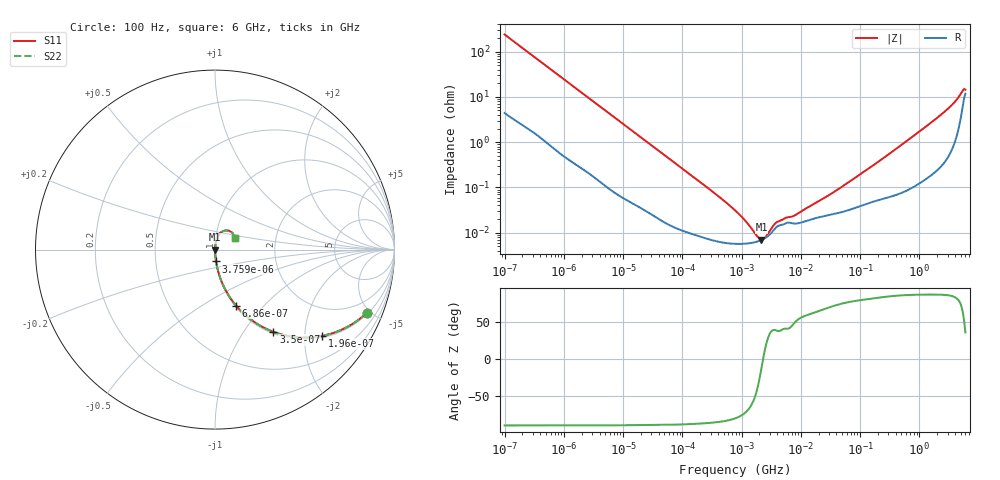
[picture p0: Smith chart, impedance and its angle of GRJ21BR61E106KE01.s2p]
!Murata Part Number: GRJ21BR61E106KE01
!These Parameters are Measured in Series Mode Connection
!Data Generated on Jun 19, 2026
!  o--ll--o
!Port1  Port2
!  o------o
!Operation Temp=25[degC], DC Bias Voltage=0[V]
!Freq. Start=100[Hz] Stop=6[GHz] 401[Steps]
# Hz S RI R 50
!Freq.(Hz) S11(Real) S11(Imag) S21(Real) S21(Imag) S12(Real) S12(Imag) S22(Real) S22(Imag)
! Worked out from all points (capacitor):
!   401 points, 100 Hz to 6 GHz, reference 50 ohm
!   read as one part in series: C = 6.67 uF near 109 Hz
!   lowest |Z| = 7.08 mohm at 2.169 MHz (marker M1)
!   series resonance near 2.31 MHz, so ESL is about 710 pH
!   S11 on the Smith chart (normalised r, x): 100 Hz: 1.09, -4.75; 196 Hz: 1.05, -2.45; 350 Hz: 1.03, -1.38; 686 Hz: 1.01, -0.71; 3.759 kHz: 1.00, -0.13; 6 GHz: 1.23, +0.17
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100  0.8451 -0.3526  0.1549 0.3526  0.1549 0.3526  0.8451 -0.3526
196  0.5976 -0.4805  0.4024 0.4805  0.4024 0.4805  0.5976 -0.4805
350  0.3256 -0.4583  0.6744 0.4583  0.6744 0.4583  0.3256 -0.4583
686  0.117 -0.3116  0.883 0.3116  0.883 0.3116  0.117 -0.3116
2008  0.0174 -0.1204  0.9826 0.1204  0.9826 0.1204  0.0174 -0.1204
3759  0.0058 -0.0658  0.9942 0.0658  0.9942 0.0658  0.0058 -0.0658
40335  0.00024 -0.00638  0.9998 0.00638  0.9998 0.00638  0.00024 -0.00638
330837  6.82e-05 -0.000789  0.9999 0.000789  0.9999 0.000789  6.82e-05 -0.000789
774597  5.71e-05 -0.000308  0.9999 0.000308  0.9999 0.000308  5.71e-05 -0.000308
1585629  6.09e-05 -9.03e-05  0.9999 9.03e-05  0.9999 9.03e-05  6.09e-05 -9.03e-05
1813585  6.36e-05 -5.74e-05  0.9999 5.74e-05  0.9999 5.74e-05  6.36e-05 -5.74e-05
2169299  6.92e-05 -1.48e-05  0.9999 1.48e-05  0.9999 1.48e-05  6.92e-05 -1.48e-05
2713602  8.2e-05 3.8e-05  0.9999 -3.8e-05  0.9999 -3.8e-05  8.2e-05 3.8e-05
4060267  0.00014 0.000107  0.9999 -0.000107  0.9999 -0.000107  0.00014 0.000107
7947587  0.000159 0.000183  0.9998 -0.000183  0.9998 -0.000183  0.000159 0.000183
1.555665e7  0.0002 0.000361  0.9998 -0.000361  0.9998 -0.000361  0.0002 0.000361
4.35672e7  0.000275 0.000887  0.9997 -0.000887  0.9997 -0.000887  0.000275 0.000887
3.124326e8  0.000643 0.00549  0.9994 -0.00549  0.9994 -0.00549  0.000643 0.00549
1.791126e9  0.00303 0.0305  0.997 -0.0305  0.997 -0.0305  0.00303 0.0305
3.666503e9  0.0121 0.0673  0.9879 -0.0673  0.9879 -0.0673  0.0121 0.0673
5.245841e9  0.0581 0.1068  0.9419 -0.1068  0.9419 -0.1068  0.0581 0.1068
6e9  0.11 0.0666  0.89 -0.0666  0.89 -0.0666  0.11 0.0666
